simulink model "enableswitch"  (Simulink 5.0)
settings: Solver=ode45  StartTime=0.0  StopTime=40.0  RelTol=1e-6

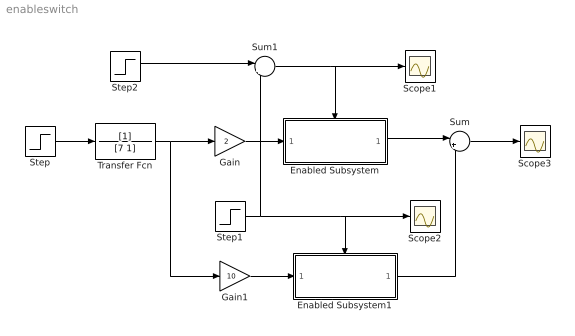
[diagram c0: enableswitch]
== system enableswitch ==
  Enabled Subsystem : Subsystem  TreatAsAtomicUnit=on
  Enabled Subsystem1 : Subsystem  TreatAsAtomicUnit=on
  Gain : Gain  Gain=2
  Gain1 : Gain  Gain=10
  Scope1 : Scope
  Scope2 : Scope
  Scope3 : Scope
  Step : Step  Time=0  SampleTime=0
  Step1 : Step  Time=20  SampleTime=0
  Step2 : Step  Time=0  SampleTime=0
  Sum : Sum  Inputs=|++
  Sum1 : Sum  Inputs=|+-
  Transfer Fcn : TransferFcn  Denominator=[7 1]
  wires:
  Sum1/1 -> Enabled Subsystem/Enable, Scope1/1
  Step1/1 -> Scope2/1, Enabled Subsystem1/Enable, Sum1/2
  Enabled Subsystem/1(Out1) -> Sum/1
  Enabled Subsystem1/1(Out1) -> Sum/2
  Sum/1 -> Scope3/1
  Gain1/1 -> Enabled Subsystem1/1(In1)
  Transfer Fcn/1 -> Gain/1, Gain1/1
  Gain/1 -> Enabled Subsystem/1(In1)
  Step/1 -> Transfer Fcn/1
  Step2/1 -> Sum1/1

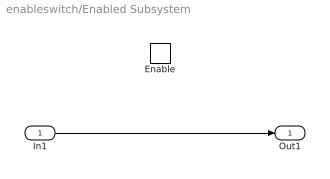
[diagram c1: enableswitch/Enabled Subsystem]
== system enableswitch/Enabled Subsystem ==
  In1 : Inport
  Enable : EnablePort
  Out1 : Outport  OutputWhenDisabled=reset  InitialOutput=[0]
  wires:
  In1/1 -> Out1/1

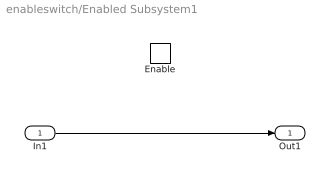
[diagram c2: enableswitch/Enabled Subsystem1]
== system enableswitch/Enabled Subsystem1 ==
  In1 : Inport
  Enable : EnablePort
  Out1 : Outport  OutputWhenDisabled=reset  InitialOutput=[0]
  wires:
  In1/1 -> Out1/1
